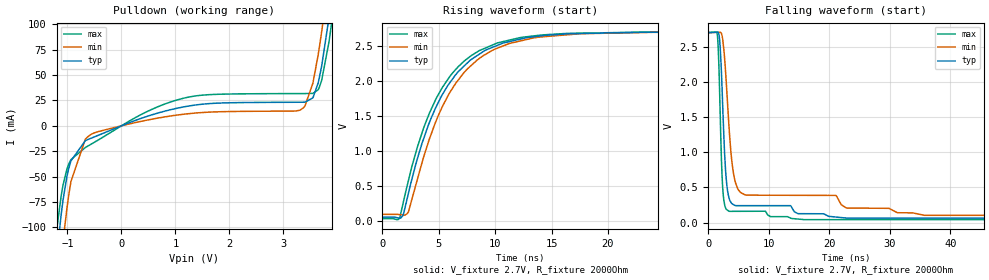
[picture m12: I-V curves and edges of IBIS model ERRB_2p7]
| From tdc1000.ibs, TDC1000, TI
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|   Model
[Model]   ERRB_2p7
Model_type   Open_drain
Polarity   Non-Inverting
Vmeas = 1.35
Vref = 2.7
Cref = 1pF
Rref = 2000
|   typ   min   max
C_comp   0.791pF   0.756pF   0.854pF
[Voltage Range]   2.7   2.699   2.701
[Temperature Range]   27   125   -40
[Pullup Reference]   2.7   2.699   2.701
[Pulldown Reference]   0   0   0
[Power Clamp Reference]   2.7   2.699   2.701
[GND Clamp Reference]   0   0   0
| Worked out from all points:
|   slope of the pulldown table from 0 to 0.405 V, typ, clamps not added: 50.2 ohm
|   falling waveform, V_fixture 2.7V, R_fixture 2000Ohm: 20-80 % time 846ps typ, 1.51ns min, 557ps max; typ from 2.7 V to 0.062 V
|   rising waveform, V_fixture 2.7V, R_fixture 2000Ohm: 20-80 % time 4.38ns typ, 4.43ns min, 4.22ns max; typ from 0.062 V to 2.7 V
[Pulldown]
|   Voltage   I(typ)   I(min)   I(max)
-2.7V     -1.097A    -1.139A    -1.07A
-1.185V   -122.1mA   -168.5mA   -97.6mA
-1.08V    -73.29mA   -113.8mA   -58.46mA
-934.2mV  -34.54mA   -54.98mA   -33.31mA
-553.5mV  -12.06mA   -8.196mA   -17.88mA
1.147V    18.57mA    11.37mA    27.14mA
3.302V    23.23mA    15.36mA    31.78mA
3.545V    27.56mA    42.05mA    31.92mA
3.707V    58.8mA     92.59mA    44.7mA
3.845V    107.1mA    148.5mA    83.17mA
3.999V    172.4mA    218.3mA    142.6mA
5.4V      890.2mA    952.3mA    838mA
[Ramp]
R_load = 2000
|   typ   min   max
dV/dt_r   1.58308/4.35074e-09   1.55839/4.42698e-09   1.59626/4.22126e-09
dV/dt_f   1.58308/8.45912e-10   1.55839/1.50907e-09   1.59626/5.57049e-10
[Falling Waveform]
V_fixture = 2.7V
V_fixture_min = 2.699V
V_fixture_max = 2.701V
R_fixture = 2000Ohm
C_fixture = 0F
|   Time   V(typ)   V(min)   V(max)
0s        2.7V       2.699V     2.701V
1.408ns   2.706V     2.704V     2.709V
1.823ns   2.65V      2.705V     2.065V
2.173ns   2.159V     2.692V     930.7mV
2.437ns   1.561V     2.574V     444.4mV
2.855ns   757.5mV    2.162V     211.9mV
3.399ns   366mV      1.413V     161.6mV
4.503ns   241.6mV    567.3mV    159.6mV
6.356ns   240mV      389.3mV    160mV
100ns     61.53mV    101.7mV    40.56mV
[Rising Waveform]
V_fixture = 2.7V
V_fixture_min = 2.699V
V_fixture_max = 2.701V
R_fixture = 2000Ohm
C_fixture = 0F
|   Time   V(typ)   V(min)   V(max)
0s        61.53mV    101.7mV    40.56mV
1.547ns   47.02mV    97.95mV    53.59mV
1.835ns   90.17mV    92.11mV    257.1mV
2.306ns   398.8mV    133.9mV    579.7mV
4.048ns   1.359V     1.115V     1.493V
5.97ns    1.974V     1.834V     2.064V
8.594ns   2.384V     2.324V     2.435V
12.22ns   2.599V     2.573V     2.621V
23.96ns   2.697V     2.696V     2.699V
100ns     2.7V       2.699V     2.701V
